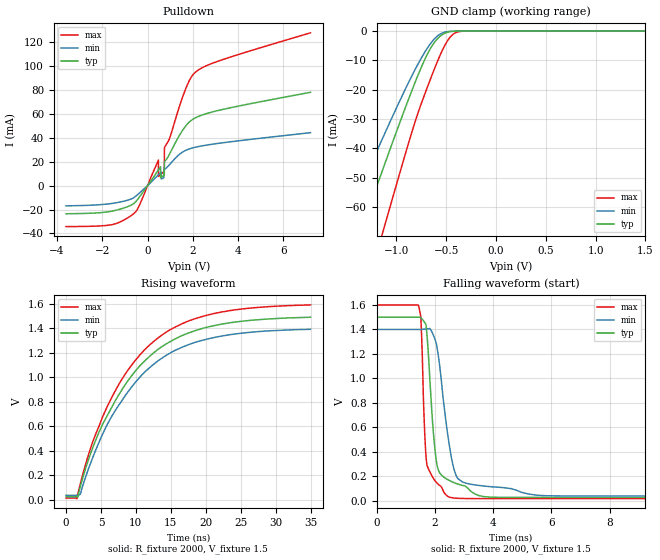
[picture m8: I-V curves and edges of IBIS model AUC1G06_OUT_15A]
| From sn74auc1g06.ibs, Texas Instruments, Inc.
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[Model]   AUC1G06_OUT_15A
Model_type  Open_drain
Enable   Active-Low
Vref =   0
Rref =   2000
Cref =   15p
Vmeas =   0.75
| variable   typ   min   max
C_comp   2.80pF   2.35pF   3.31pF
| C_pulldown   3.81pF   3.31pF   4.46pF
| C_tri-state   2.80pF   2.35pF   3.31pF
[Temperature Range]   40   100   -40
| Ambient temperature   25   85   -40
[Voltage range]   1.5   1.4   1.6
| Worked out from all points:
|   slope of the pulldown table from 0 to 0.225 V, typ, clamps not added: 37.3 ohm
|   GND clamp passes 1 mA (typ) near -0.53 V on its own axis
|   rising waveform, R_fixture 2000, V_fixture 1.5: 20-80 % time 9.33ns typ, 9.3ns min, 9.19ns max; typ from 0.027 V to 1.49 V
|   falling waveform, R_fixture 2000, V_fixture 1.5: 20-80 % time 277ps typ, 451ps min, 152ps max; typ from 1.5 V to 0.027 V
[GND Clamp]
| AUC1G06_OUT_15A
|   Voltage   I(typ)   I(min)   I(max)
-3.6V     -288.1mA   -237.2mA   -357.2mA
-1.54V    -85.96mA   -67.71mA   -116.4mA
-1.355V   -68.01mA   -53.14mA   -94.44mA
-1.165V   -49.79mA   -38.5mA    -71.85mA
-1.115V   -45.05mA   -34.73mA   -65.91mA
-835mV    -19.39mA   -14.59mA   -33.3mA
-690mV    -7.898mA   -5.836mA   -19.16mA
-565mV    -1.877mA   -1.115mA   -8.49mA
-490mV    -444.9uA   -218.1uA   -3.452mA
-430mV    -100.1uA   -52.71uA   -1.068mA
-305mV    -2.545uA   -2.112uA   -19.74uA
1.5V      322pA      495.8pA    331.6pA
[Pulldown]
| AUC1G06_OUT_15A
|   Voltage   I(typ)   I(min)   I(max)
-3.6V     -23.47mA   -16.88mA   -34.23mA
-1.535V   -21.16mA   -14.74mA   -32.45mA
-520mV    -13.36mA   -8.761mA   -21.72mA
480mV     13.33mA    9.224mA    21.44mA
485mV     13.46mA    9.315mA    7.619mA
720mV     8.537mA    6.728mA    11.81mA
735mV     8.725mA    13.4mA     12.06mA
745mV     18.83mA    13.55mA    29.66mA
760mV     20.34mA    13.77mA    32.32mA
1.73V     51.03mA    29.96mA    83.16mA
2.16V     57.24mA    32.41mA    95.72mA
7.2V      78.21mA    44.4mA     128mA
[Ramp]
| AUC1G06_OUT_15A
| variable   typ   min   max
dV/dt_r   0.88/9.35E-09   0.81/9.30E-09   0.95/9.19E-09
dV/dt_f   0.88/2.94E-10   0.82/4.72E-10   0.95/1.63E-10
R_load = 2000
[Rising Waveform]
| AUC1G06_OUT_15A
R_fixture =   2000
C_fixture =   0
L_fixture =   0
V_fixture =   1.5
V_fixture_min = 1.4
V_fixture_max = 1.6
|   Time   V(typ)   V(min)   V(max)
0s        27.17mV    38.78mV    16.4mV
1.555ns   26.41mV    38.88mV    10.93mV
2.055ns   110.4mV    49.24mV    135.5mV
3.86ns    431.5mV    351.4mV    479.6mV
7.445ns   847.1mV    763.4mV    930.3mV
10.11ns   1.064V     971.2mV    1.151V
12.95ns   1.218V     1.124V     1.31V
16.67ns   1.341V     1.245V     1.437V
21.03ns   1.418V     1.322V     1.517V
34.99ns   1.489V     1.391V     1.589V
[Falling Waveform]
| AUC1G06_OUT_15A
R_fixture =   2000
C_fixture =   0
L_fixture =   0
V_fixture =   1.5
V_fixture_min = 1.4
V_fixture_max = 1.6
|   Time   V(typ)   V(min)   V(max)
0s        1.5V       1.4V       1.6V
1.43ns    1.5V       1.4V       1.601V
1.52ns    1.495V     1.4V       1.494V
1.645ns   1.459V     1.402V     599.3mV
1.73ns    1.357V     1.405V     292.8mV
2.06ns    313.4mV    1.275V     148.6mV
2.575ns   156.3mV    345.7mV    24.44mV
2.975ns   123.3mV    150.7mV    18.11mV
5.84ns    27.11mV    40.2mV     16.36mV
34.99ns   27.17mV    38.78mV    16.4mV
